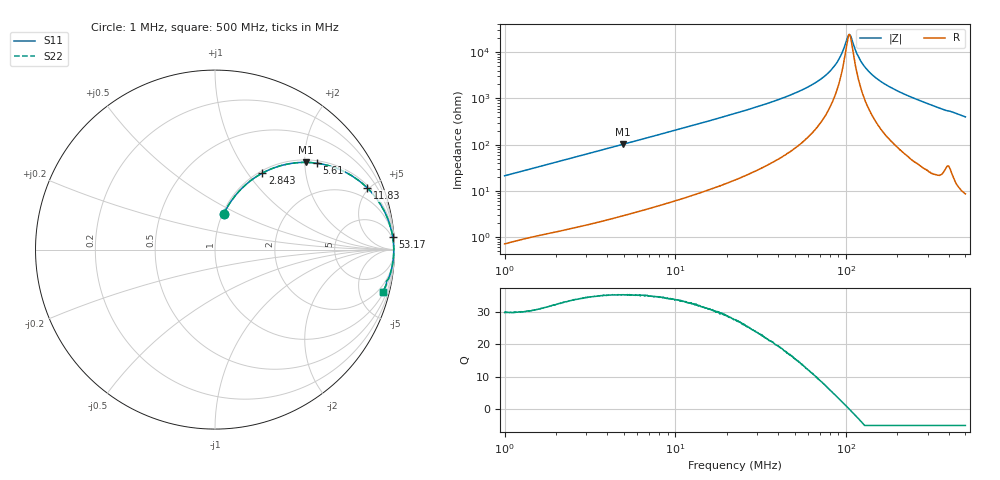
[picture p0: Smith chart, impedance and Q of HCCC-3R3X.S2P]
!s-Parameter Generated by FASTRON Sdn. Bhd.
!FASTRON P/N : HCCC-3R3X
!Keysight Technologies,E4991B,MY54100416,A.01.15
!Date: Thu Apr 02 14:28:24 2026
!Version  : Rev00 Thu Apr 02 14:28:24 2026
!Data & Calibration Information:
!PortZ  Port1:50+j0  Port2:50+j0
!When reading, reference impedance value at option line is always used.
! Remarks : This data is being provided solely for informational purposes.
!Freq	S11	S21	S12	S22
# Hz S dB R 50
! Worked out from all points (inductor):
!   1601 points, 1 MHz to 500 MHz, reference 50 ohm
!   read as one part in series: L = 3.35 uH near 1.032 MHz
!   highest Q = 35.2 at 4.935 MHz (marker M1), where L = 3.27 uH
!   self-resonance near 104.1 MHz
!   S11 on the Smith chart (normalised r, x): 1 MHz: 1.01, +0.42; 2.843 MHz: 1.03, +1.18; 5.61 MHz: 1.07, +2.30; 11.83 MHz: 1.15, +4.85; 53.17 MHz: 3, +28; 500 MHz: 1.17, -7.95
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1000000  -13.73 76.2  -0.25 -11.9  -0.25 -11.9  -13.73 76.2
2820919  -6.05 58.4  -1.39 -29.9  -1.39 -29.9  -6.05 58.4
2842918  -6.00 58.3  -1.40 -30.1  -1.40 -30.1  -6.00 58.3
4935122  -3.07 43.8  -3.20 -44.6  -3.20 -44.6  -3.07 43.8
5610017  -2.56 40.2  -3.79 -48.1  -3.79 -48.1  -2.56 40.2
7957584  -1.50 31.1  -5.75 -57.3  -5.75 -57.3  -1.50 31.1
1.182607e7  -0.77 22.1  -8.48 -66.1  -8.48 -66.1  -0.77 22.1
2.236068e7  -0.26 11.9  -13.72 -76.0  -13.72 -76.0  -0.26 11.9
5.316844e7  -0.06 4.0  -23.14 -82.1  -23.14 -82.1  -0.06 4.0
6.307767e7  -0.05 2.9  -25.91 -81.9  -25.91 -81.9  -0.05 2.9
7.483371e7  -0.04 1.9  -29.63 -80.6  -29.63 -80.6  -0.04 1.9
8.506748e7  -0.04 1.1  -33.81 -76.9  -33.81 -76.9  -0.04 1.1
9.229699e7  -0.04 0.7  -37.89 -69.8  -37.89 -69.8  -0.04 0.7
1.017089e8  -0.04 0.1  -46.21 -32.2  -46.21 -32.2  -0.04 0.1
1.045122e8  -0.04 -0.0  -47.67 0.1  -47.67 0.1  -0.04 -0.0
1.073927e8  -0.04 -0.1  -46.22 32.0  -46.22 32.0  -0.04 -0.1
1.18344e8  -0.04 -0.7  -37.90 70.5  -37.90 70.5  -0.04 -0.7
1.294029e8  -0.04 -1.2  -33.45 77.8  -33.45 77.8  -0.04 -1.2
1.476717e8  -0.04 -2.0  -29.21 81.4  -29.21 81.4  -0.04 -2.0
1.77937e8  -0.05 -3.1  -25.22 82.6  -25.22 82.6  -0.05 -3.1
2.685796e8  -0.09 -6.3  -19.22 81.4  -19.22 81.4  -0.09 -6.3
5e8  -0.31 -14.0  -12.29 74.7  -12.29 74.7  -0.31 -14.0
